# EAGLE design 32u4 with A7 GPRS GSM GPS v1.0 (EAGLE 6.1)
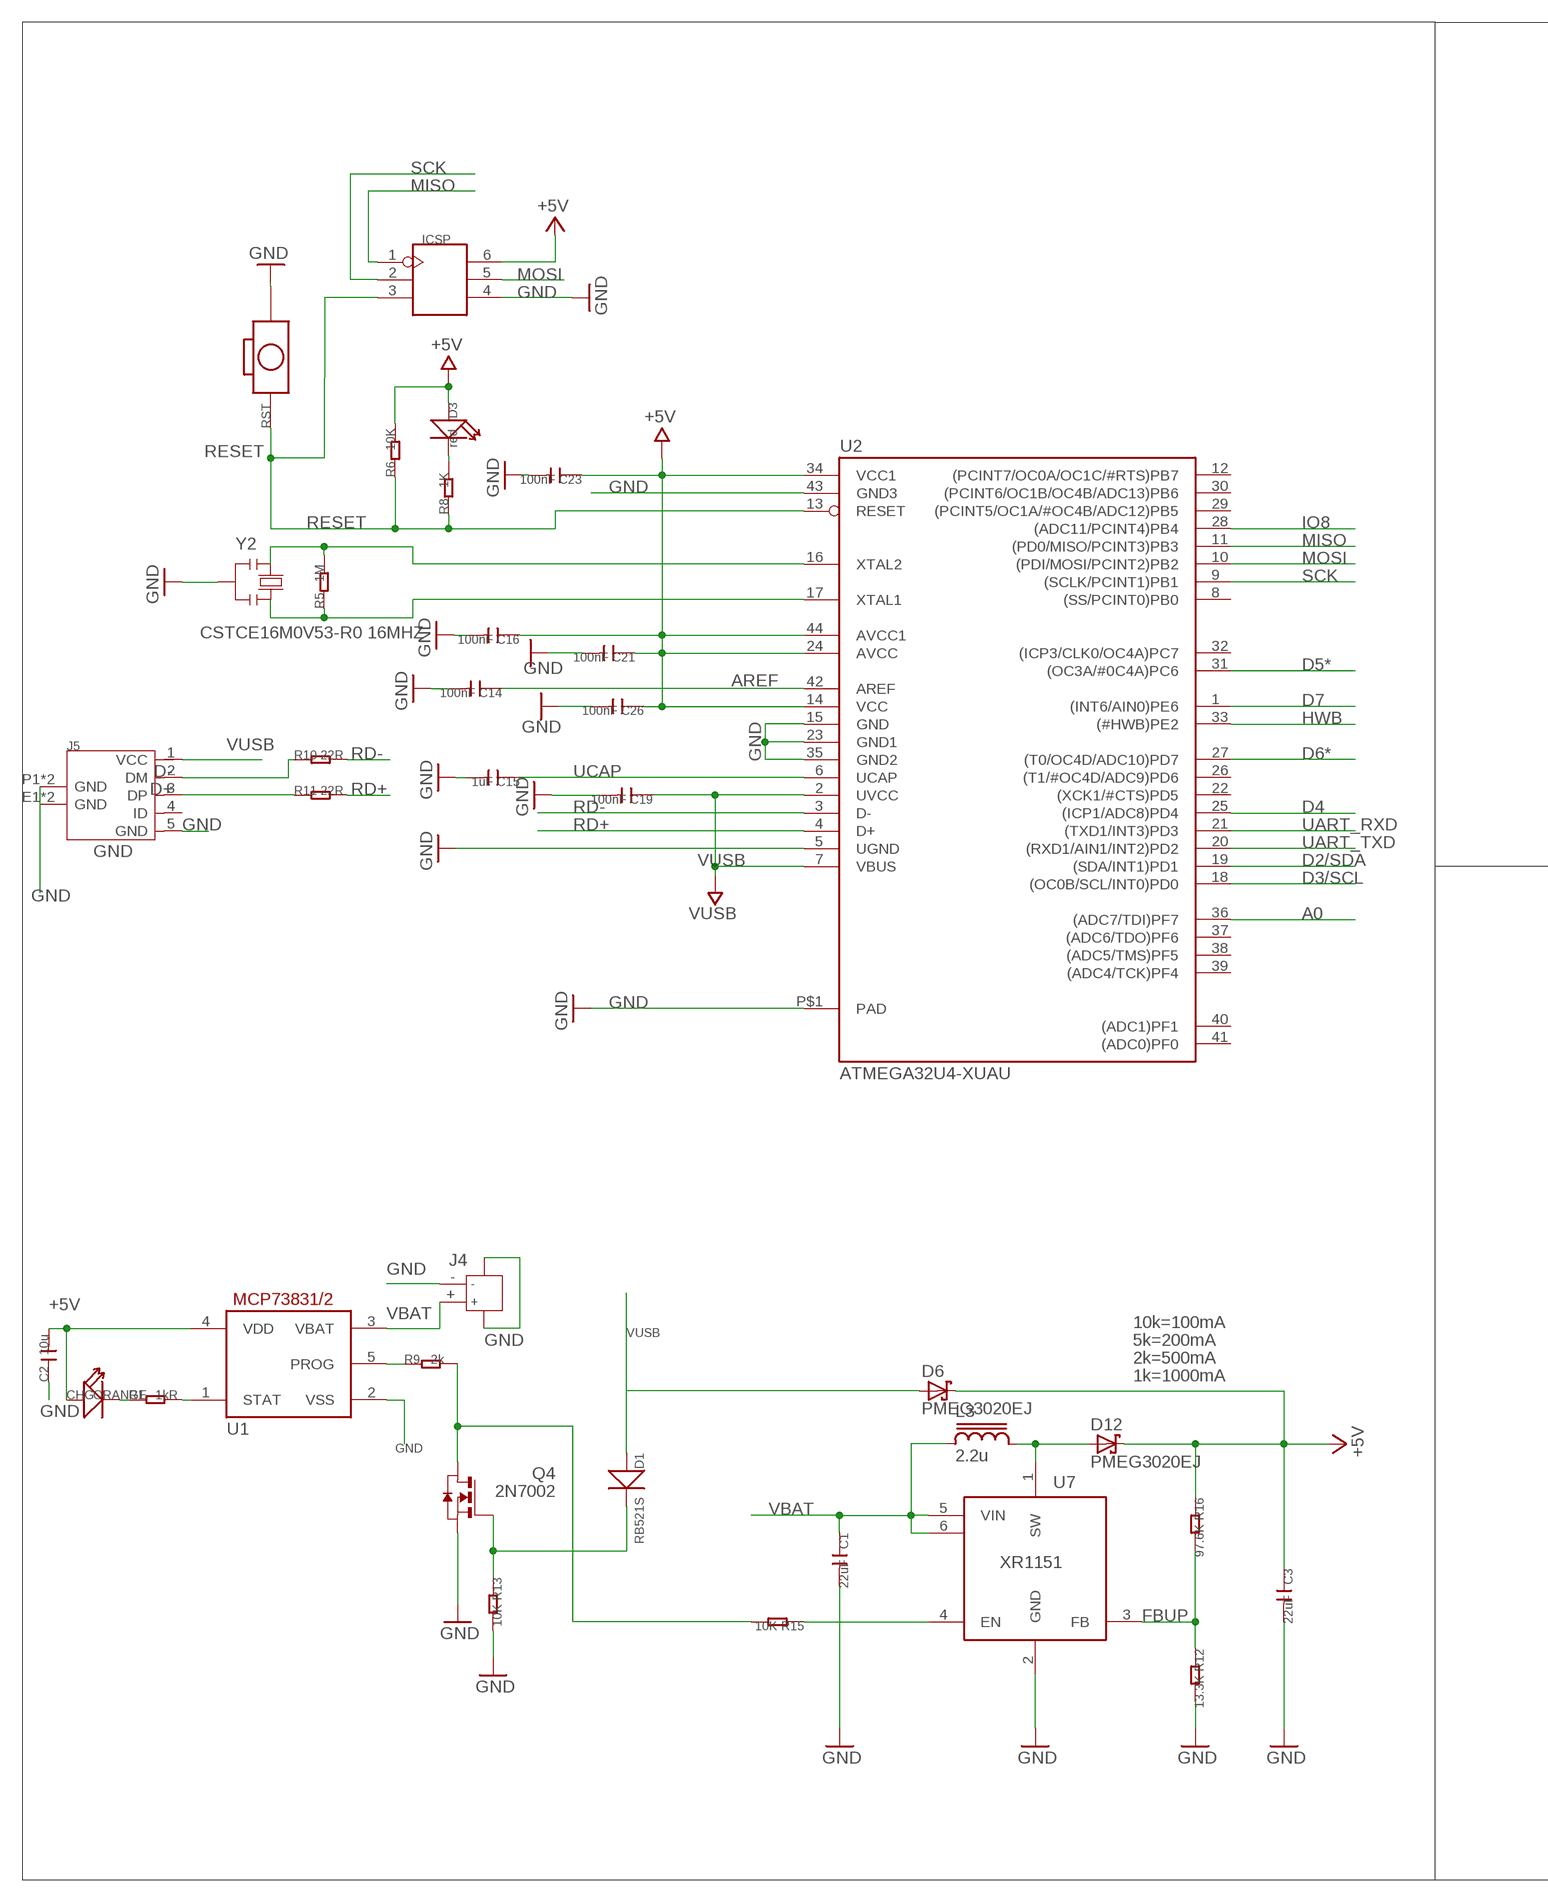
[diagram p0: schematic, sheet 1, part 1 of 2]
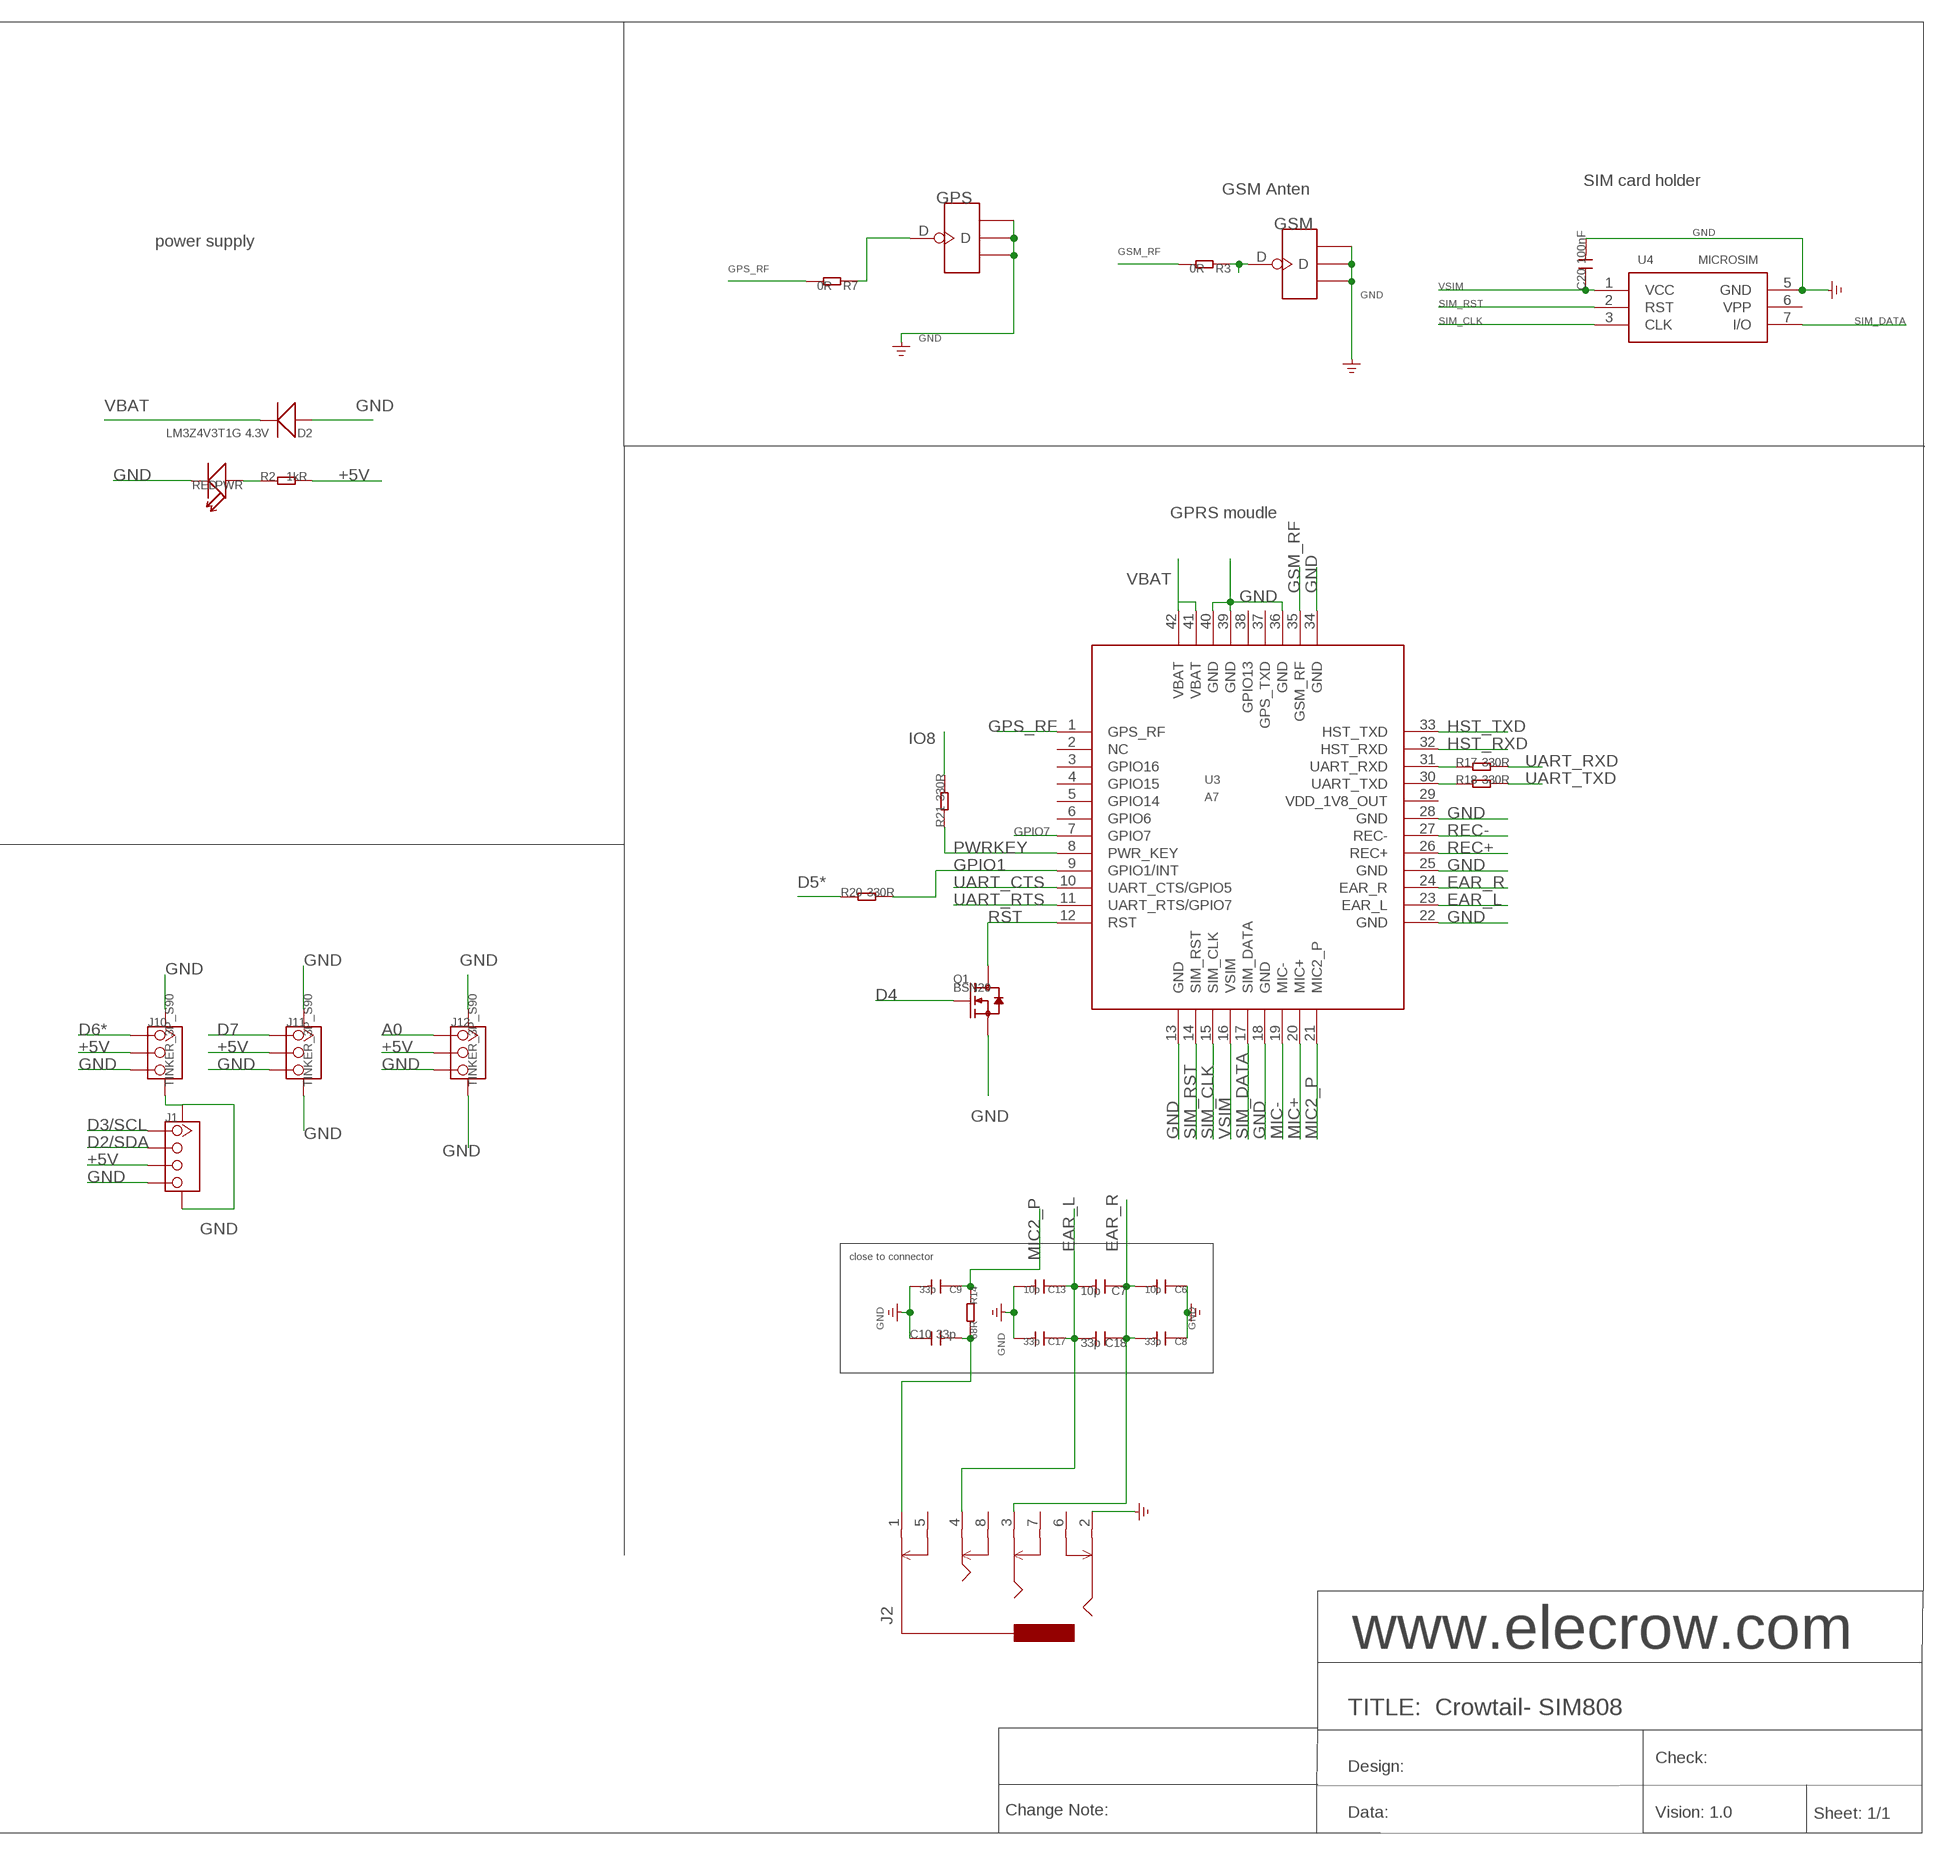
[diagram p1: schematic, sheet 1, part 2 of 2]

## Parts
C1  22uF  C-0603  [C0603]
C2  10u  C-0603  [C0603]
C3  22uF  C-0603  [C0603]
C6  10p  C-0402  [C0402]
C7  10p  C-0402  [C0402]
C8  33p  C-0402  [C0402]
C9  33p  C-0603  [C0603]
C10  33p  C-0603  [C0603]
C13  10p  C-0402  [C0402]
C14  100nF  C-0603  [C0603]
C15  1uF  C-0603  [C0603]
C16  100nF  C-0603  [C0603]
C17  33p  C-0402  [C0402]
C18  33p  C-0402  [C0402]
C19  100nF  C-0603  [C0603]
C20  100nF  C-0603  [C0603]
C21  100nF  C-0603  [C0603]
C23  100nF  C-0603  [C0603]
C26  100nF  C-0603  [C0603]
CHG  ORANGE  007-LED0603  [D0603]
D1  RB521S  D'0603'  [SOD523]
D2  LM3Z4V3T1G 4.3V  D'0805'  [SOD323]
D3  red  LED'0603'  [LED-0603]
D6  PMEG3020EJ  [SOD-323]
D12  PMEG3020EJ  [SOD-323]
GPS  ANTENNA-U-FL  [4P-U-FL]
GSM  ANTENNA-U-FL  [4P-U-FL]
ICSP  HEADER-2X3P-2.0  [2X3P-2.0]
J1  TWIG-4P-2.0-SMD-FEMALE-REINFORCE'90D'  [4P-SMD-2.0-90D]
J2  AUDIO-8P'PJ-3536-L6S'  [8P-3.5-SMD]
J4  JACK-JST-2P-SMD-PW'2.0'  [JST-SMD-2.0-90D]
J5  MICRO-USB-5P-340015001  [B-SMD-5P]
J10  TINKER_3P_S90  [TINKER_3P_S90]
J11  TINKER_3P_S90  [TINKER_3P_S90]
J12  TINKER_3P_S90  [TINKER_3P_S90]
L3  2.2u  LCD32  [CD32]
PWR  RED  007-LED0603  [D0603]
Q1  BSN20  MOSFET-N'SOT23'  [SOT23@1]
Q4  2N7002  [SOT23]
R1  1kR  R-0603  [R0603]
R2  1kR  R-0603  [R0603]
R3  0R  R-0603  [R0603]
R5  1M  R-0603  [R0603]
R6  10K  R-0603  [R0603]
R7  0R  R-0603  [R0603]
R8  1K  R-0603  [R0603]
R9  2k  R-0603  [R0603]
R10  22R  R-0603  [R0603]
R11  22R  R-0603  [R0603]
R12  13.3K  R-0603  [R0603]
R13  10K  R-0603  [R0603]
R14  68R  R-0603  [R0603]
R15  10K  R-0603  [R0603]
R16  97.6K  R-0603  [R0603]
R17  330R  R-0603  [R0603]
R18  330R  R-0603  [R0603]
R20  330R  R-0603  [R0603]
R21  330R  R-0603  [R0603]
RST  BOTTON-2P-90D  [2P-7.62X3.56-90D]
U1  MCP73831/OT  [SOT23-5L]
U2  ATMEGA32U4-XUAU  [TQFP44-PAD]
U3  A7  [A7]
U4  MICROSIM  [MICROSIM]
U7  XR1151  [SOT23-6L]
Y2  CSTCE16M0V53-R0 16MHZ  RESONATORMU  [RESONATOR]

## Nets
+5V: C2.2 C3.1 C16.1 C21.1 C23.1 C26.1 CHG.+ D3.+ D6.C D12.C ICSP.6 J1.3 J10.2 J11.2 J12.2 R2.2 R6.2 R16.1 U1.4(VDD) U2.14(VCC) U2.24(AVCC) U2.34(VCC1) U2.44(AVCC1)
A0: J12.1 U2.36((ADC7/TDI)PF7)
AREF [aref]: C14.1 U2.42(AREF)
D2/SDA: J1.2 U2.19((SDA/INT1)PD1)
D3/SCL: J1.1 U2.18((OC0B/SCL/INT0)PD0)
D4: Q1.1(G) U2.25((ICP1/ADC8)PD4)
D5*: R20.1 U2.31((OC3A/#0C4A)PC6)
D6*: J10.1 U2.27((T0/OC4D/ADC10)PD7)
D7: J11.1 U2.1((INT6/AIN0)PE6)
D+: J5.3(DP) R11.1
D-: J5.2(DM) R10.1
EAR_L: C7.2 C13.1 C17.1 C18.2 J2.4 U3.23(EAR_L)
EAR_R: C6.2 C7.1 C8.2 C18.1 J2.3 U3.24(EAR_R)
FBUP: R12.1 R16.2 U7.3(FB)
GND: C1.2 C2.1 C3.2 C6.1 C8.1 C9.2 C10.1 C13.2 C14.2 C15.2 C16.2 C17.2 C19.2 C20.2 C21.2 C23.2 C26.2 D2.+ GPS.GND1 GPS.GND2 GPS.GND3 GSM.GND1 GSM.GND2 GSM.GND3 ICSP.4 J1.4 J1.SS1 J1.SS2 J2.2 J4.3 J4.4 J4.- J5.5(GND) J5.E1(GND) J5.E2(GND) J5.P1(GND) J5.P2(GND) J10.3 J10.SS1 J10.SS2 J11.3 J11.SS1 J11.SS2 J12.3 J12.SS1 J12.SS2 PWR.- Q1.2(S) Q4.2(S) R12.2 R13.2 RST.P$2 U1.2(VSS) U2.5(UGND) U2.15(GND) U2.23(GND1) U2.35(GND2) U2.43(GND3) U2.P$1(PAD) U3.13(GND) U3.18(GND) U3.22(GND) U3.25(GND) U3.28(GND) U3.34(GND) U3.36(GND) U3.39(GND) U3.40(GND) U4.5(GND) U7.2(GND) Y2.2
GPIO1: R20.2 U3.9(GPIO1/INT)
GPIO7: U3.7(GPIO7)
GPS_RF: R7.2 U3.1(GPS_RF)
GSM_RF: R3.2 U3.35(GSM_RF)
HST_RXD: U3.32(HST_RXD)
HST_TXD: U3.33(HST_TXD)
HWB: U2.33((#HWB)PE2)
IO8: R21.2 U2.28((ADC11/PCINT4)PB4)
MIC2_P: C9.1 R14.1 U3.21(MIC2_P)
MIC+: U3.20(MIC+)
MIC-: U3.19(MIC-)
MISO: ICSP.1 U2.11((PD0/MISO/PCINT3)PB3)
MOSI: ICSP.5 U2.10((PDI/MOSI/PCINT2)PB2)
N$1: D12.A L3.2 U7.1(SW)
N$2: Q4.3(D) R9.2 R15.2
N$3: D1.- Q4.1(G) R13.1
N$4: R17.1 U3.31(UART_RXD)
N$5: GSM.D R3.1
N$6: PWR.+ R2.1
N$7: GPS.D R7.1
N$10: R15.1 U7.4(EN)
N$11: CHG.- R1.1
N$14: R18.1 U3.30(UART_TXD)
N$15: D3.- R8.2
N$20: R1.2 U1.1(STAT)
N$30: C10.2 J2.1 R14.2
N$31: R9.1 U1.5(PROG)
PWRKEY: R21.1 U3.8(PWR_KEY)
RD+: R11.2 U2.4(D+)
RD-: R10.2 U2.3(D-)
REC+: U3.26(REC+)
REC-: U3.27(REC-)
RESET: ICSP.3 R6.1 R8.1 RST.P$1 U2.13(RESET)
RST: Q1.3(D) U3.12(RST)
SCK: ICSP.2 U2.9((SCLK/PCINT1)PB1)
SIM_CLK: U3.15(SIM_CLK) U4.3(CLK)
SIM_DATA: U3.17(SIM_DATA) U4.7(I/O)
SIM_RST: U3.14(SIM_RST) U4.2(RST)
UART_CTS: U3.10(UART_CTS/GPIO5)
UART_RTS: U3.11(UART_RTS/GPIO7)
UART_RXD: R17.2 U2.21((TXD1/INT3)PD3)
UART_TXD: R18.2 U2.20((RXD1/AIN1/INT2)PD2)
UCAP: C15.1 U2.6(UCAP)
VBAT: C1.1 D2.- J4.+ L3.1 U1.3(VBAT) U3.41(VBAT) U3.42(VBAT) U7.5(VIN) U7.6(VIN1)
VSIM: C20.1 U3.16(VSIM) U4.1(VCC)
VUSB: C19.1 D1.+ D6.A J5.1(VCC) U2.2(UVCC) U2.7(VBUS)
XTAL3: R5.2 U2.16(XTAL2) Y2.1
XTAL4: R5.1 U2.17(XTAL1) Y2.3
Unconnected: J2.5 J2.6 J2.7 J2.8 J5.4(ID) U2.8((SS/PCINT0)PB0) U2.12((PCINT7/OC0A/OC1C/#RTS)PB7) U2.22((XCK1/#CTS)PD5) U2.26((T1/#OC4D/ADC9)PD6) U2.29((PCINT5/OC1A/#OC4B/ADC12)PB5) U2.30((PCINT6/OC1B/OC4B/ADC13)PB6) U2.32((ICP3/CLK0/OC4A)PC7) U2.37((ADC6/TDO)PF6) U2.38((ADC5/TMS)PF5) U2.39((ADC4/TCK)PF4) U2.40((ADC1)PF1) U2.41((ADC0)PF0) U3.2(NC) U3.3(GPIO16) U3.4(GPIO15) U3.5(GPIO14) U3.6(GPIO6) U3.29(VDD_1V8_OUT) U3.37(GPS_TXD) U3.38(GPIO13) U4.6(VPP)

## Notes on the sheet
- SIM card holder
- GSM Anten
- power supply
- GPRS moudle
- close to connector
- 10k=100mA
- 5k=200mA
- 2k=500mA
- 1k=1000mA
- www.elecrow.com
- TITLE:  Crowtail- SIM808
- Check:
- Design:
- Change Note: | Data: | Vision: 1.0 | Sheet: 1/1

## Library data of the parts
C1-C3 C6-C10 C13-C21 C23 C26 = Discrete:C*: Ceramic Capacitors
CHG PWR = Discrete:007-LED*
D1 D2 = Discrete:D*
D3 = Discrete:LED*
D6 D12 = Max-Diodes:PMEG3020
GPS GSM = Connector:ANTENNA-U-FL
ICSP = Connector:HEADER-2X3P
J1 = Connector:TWIG-4P-2.0-SMD-FEMALE-REINFORCE
J2 = template:AUDIO-8P
J4 = Connector:JACK-JST-2P-SMD-PW
J5 = OPL Eagle Library:MICRO-USB-5P: ST-USB-001E：MICRO USB B SMD R/A
J10-J12 = Connector:TINKER_3P_S90
L3 = Max-RCL:L
Q1 = Discrete:MOSFET-N: IRLL014: http://www.vishay.com/docs/91319/sihll014.pdf
Q4 = Max-Mosfets:2N7002
R1-R3 R5-R18 R20 R21 = Discrete:R*
RST = Discrete:BOTTON-2P
U1 = adafruit:MCP73831: MCP73831/2 Miniature Single-Cell, Fully Integrated Li-Ion, Li-Polymer Charge Management Controllers. Nice and small simple lipoly charge controller, with adjustable current and status output (LED) http://www.ladyada.net/library/pcb/eaglelibrary.html
U2 = SmartPrj:ATMEGA32U4-XU
U3 = IC:A7
U4 = Connector:MICROSIM
U7 = Max-SwitchingRegulators:XR1151
Y2 = SmartPrj:RESONATOR

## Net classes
0 default: width 0.152 mm, drill 0.152 mm, clearance 0.152 mm
1 power: width 0.61 mm, drill 0.61 mm, clearance 0.203 mm
2 gnd: width 0.305 mm, drill 0.559 mm, clearance 0.203 mm
3 usbvcc: width 0.508 mm, drill 0.61 mm, clearance 0.203 mm
4 aref: width 0.254 mm, drill 0.61 mm, clearance 0.254 mm

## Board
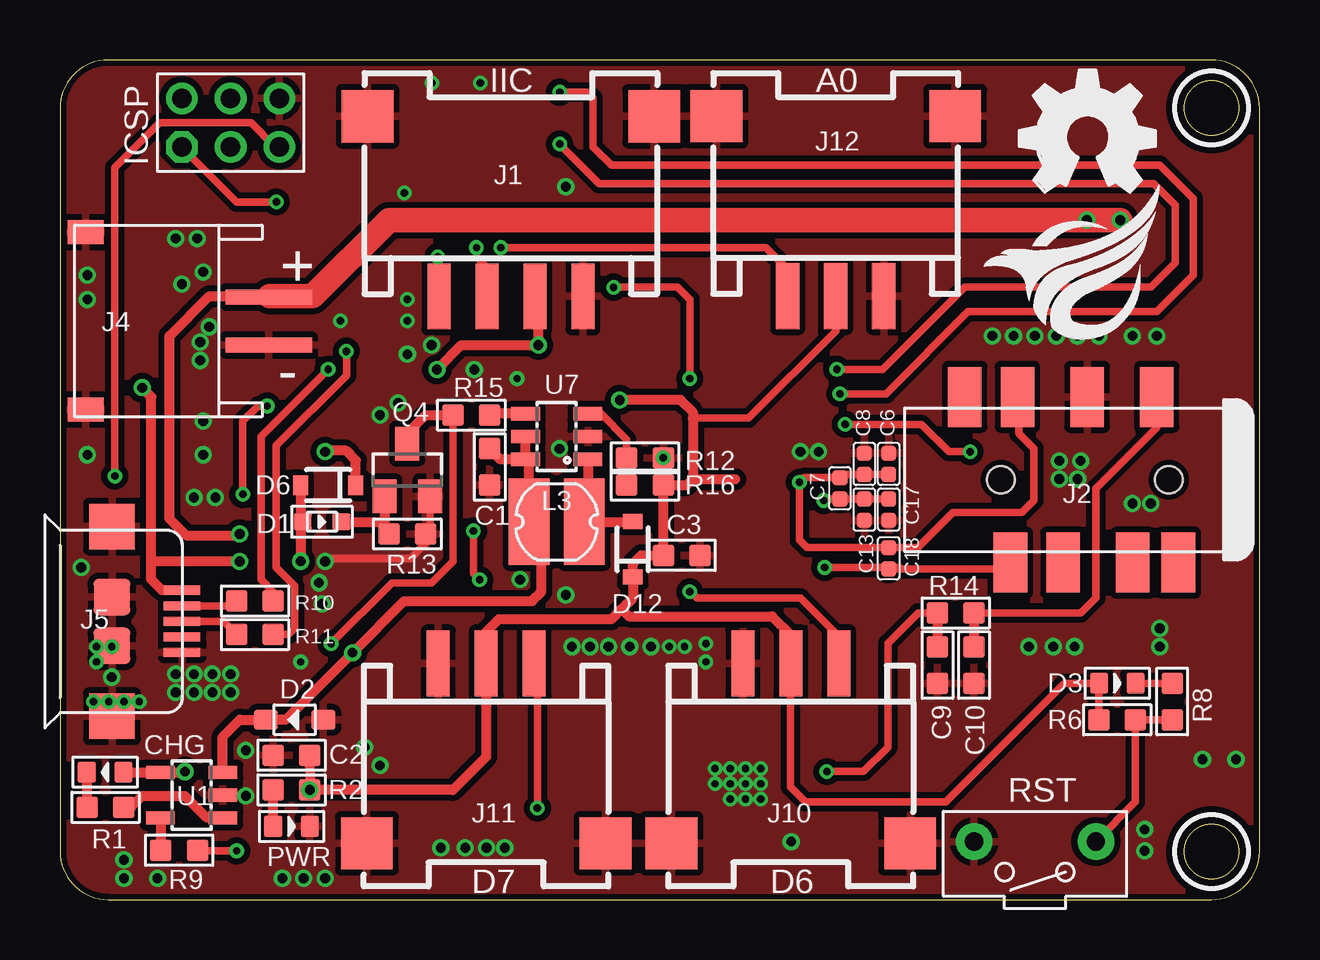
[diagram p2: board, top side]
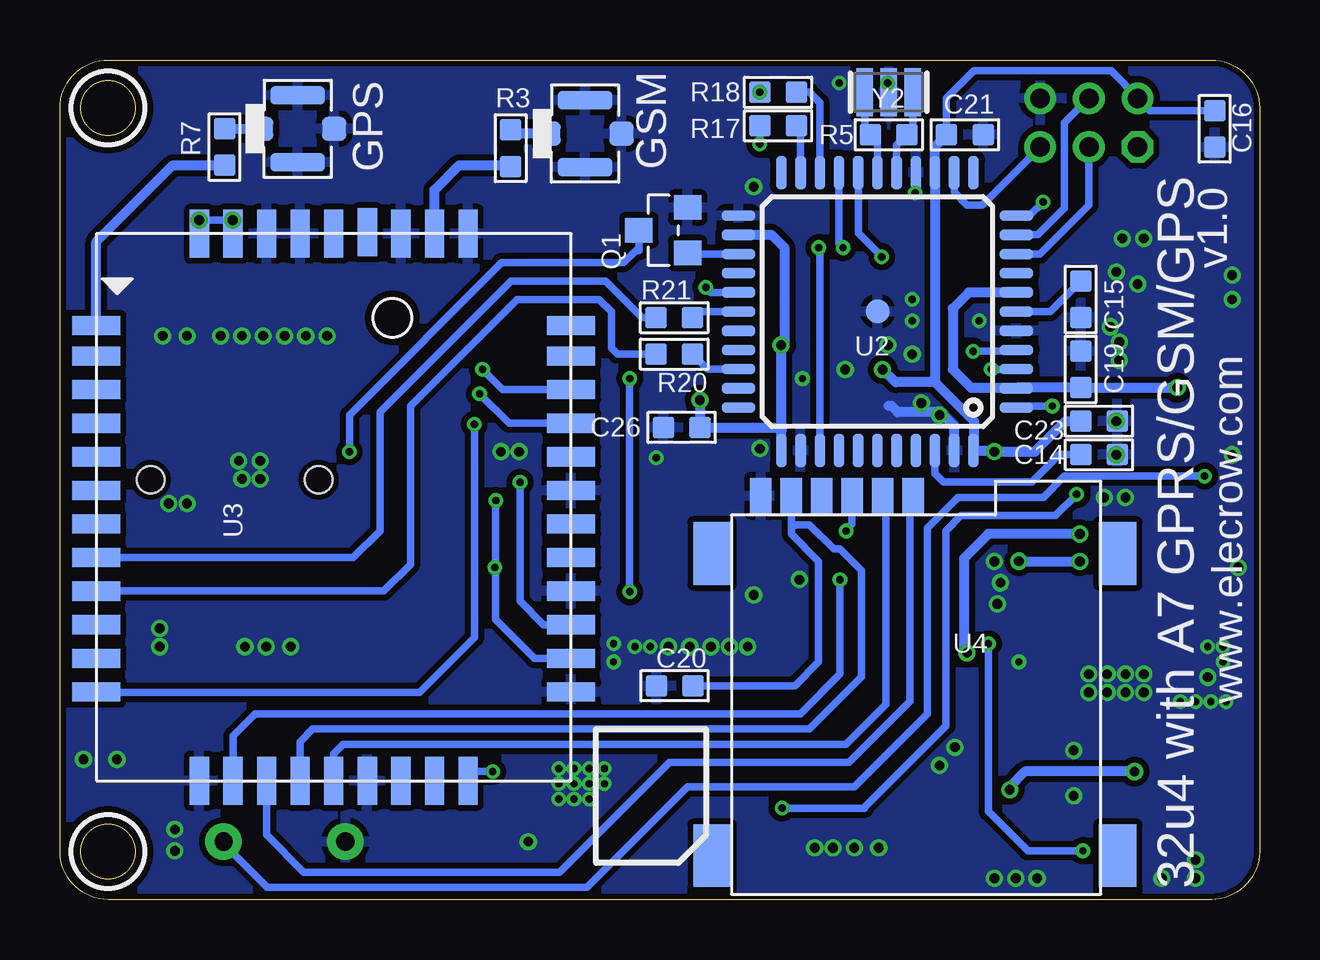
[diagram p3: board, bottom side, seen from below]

Size 50 x 35 mm. Coordinates in mm from the lower left corner, seen from the top.
Outline: 0,33 0,2 arc90 2,0 48,0 arc90 50,2 50,33 arc90 48,35 2,35 arc90 0,33
Outline: circle at 48,2 radius 1.14
Outline: circle at 48,33 radius 1.14
Copper layers (1*16): Top 0.035mm / dielectric 1.5mm / Bottom 0.035mm
Design rules: minimum track width 6mil, minimum drill 12mil, track to track 6mil, track to pad 6mil, pad to pad 6mil, via to via 6mil, smd to smd 0mil, copper to edge 10mil, drill to drill 10mil, minimum pad ring 10mil, minimum via ring 6mil, stop-mask expansion 2mil, vias tented up to drill 100mil, thermal gap 10mil
tRestrict: area 35.6,41.9 to 35.7,43.3; area 46.5,0.5 to 49.5,3.5; area 46.5,31.5 to 49.5,34.5
bRestrict: area 46.5,0.5 to 49.5,3.5; area 46.5,31.5 to 49.5,34.5

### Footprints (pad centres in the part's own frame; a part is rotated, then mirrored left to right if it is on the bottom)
C0603 = smd 0.889 x 0.889: 1 -0.762,0; 2 0.762,0
C0402 = smd 0.635 x 0.635: 1 -0.445,0; 2 0.445,0
D0603 = smd 0.762 x 0.889: + -0.762,0; - 0.762,0
SOD523 = smd 0.762 x 0.7: + -0.8,0; - 0.8,0
SOD323 = smd 1 x 0.8: + -1.2,0; - 1.2,0
LED-0603 = smd 0.762 x 0.889: + -0.762,0; - 0.762,0
SOD-323 = smd 0.63 x 0.83: A 1.15,0; C -1.15,0
4P-U-FL = smd 1.016 x 1.016: D -1.524,0; GND3 1.524,0 | smd 2.286 x 0.762: GND1 0,1.397; GND2 0,-1.397
2X3P-2.0 = drill 0.813 pad 1.27 octagon: 1 -1.016,2.032 | drill 0.813 pad 1.27: 2 -1.016,0; 3 -1.016,-2.032; 4 1.016,-2.032; 5 1.016,0; 6 1.016,2.032
4P-SMD-2.0-90D = smd 0.965 x 2.74: 1 -3,-0.1; 2 -1,-0.1; 3 1,-0.1; 4 3,-0.1 | smd 2.159 x 2.184: SS1 -5.974,7.4; SS2 5.974,7.4
8P-3.5-SMD = smd 1.4 x 2.5: 1 2.8,-3.45; 2 5.7,-3.45; 3 8.6,-3.45; 4 8.9,3.45; 5 1.9,3.45; 6 3.8,3.45; 7 6.7,3.45; 8 10.8,-3.45 | hole 1.149: 2.3,0; 9.3,0
JST-SMD-2.0-90D = smd 1 x 1.5: 3 3.7,-2.54; 4 -3.7,-2.54 | smd 0.635 x 3.6: + -1,5.08; - 1,5.08
B-SMD-5P = smd 0.38 x 1.52: 1 -1.3,2.54; 2 -0.65,2.54; 3 0,2.54; 4 0.65,2.54; 5 1.3,2.54 | smd 1.524 x 1.524: E1 -1.016,-0.381; E2 1.016,-0.381 | smd 1.9 x 1.9: P1 -3.95,-0.381; P2 3.95,-0.381
TINKER_3P_S90 = smd 0.965 x 2.74: 1 -1.984,-4.545; 2 0.016,-4.545; 3 2.016,-4.545 | smd 2.159 x 2.184: SS1 -4.958,2.955; SS2 4.99,2.955
CD32 = smd 3.6 x 1.7: 1 0,1.15; 2 0,-1.15
SOT23@1 = smd 1.016 x 1.143: 1 -0.95,-1.016; 2 0.95,-1.016; 3 0,1.016
SOT23 = smd 1 x 1.4: 1 -0.95,-1.1; 2 0.95,-1.1; 3 0,1.1
R0603 = smd 0.889 x 0.889: 1 -0.762,0; 2 0.762,0
2P-7.62X3.56-90D = drill 0.762 pad 1.524: P$1 0,2.54; P$2 0,-2.54
SOT23-5L = smd 0.55 x 1.2: 1 -0.95,-1.3; 2 0,-1.3; 3 0.95,-1.3; 4 0.95,1.3; 5 -0.95,1.3
TQFP44-PAD = smd 1.4 x 0.45: 1 -5.8,4; 2 -5.8,3.2; 3 -5.8,2.4; 4 -5.8,1.6; 5 -5.8,0.8; 6 -5.8,0; 7 -5.8,-0.8; 8 -5.8,-1.6; 9 -5.8,-2.4; 10 -5.8,-3.2; 11 -5.8,-4; 23 5.8,-4; 24 5.8,-3.2; 25 5.8,-2.4; 26 5.8,-1.6; 27 5.8,-0.8; 28 5.8,0; 29 5.8,0.8; 30 5.8,1.6; 31 5.8,2.4; 32 5.8,3.2; 33 5.8,4 | smd 0.45 x 1.4: 12 -4,-5.8; 13 -3.2,-5.8; 14 -2.4,-5.8; 15 -1.6,-5.8; 16 -0.8,-5.8; 17 0,-5.8; 18 0.8,-5.8; 19 1.6,-5.8; 20 2.4,-5.8; 21 3.2,-5.8; 22 4,-5.8; 34 4,5.8; 35 3.2,5.8; 36 2.4,5.8; 37 1.6,5.8; 38 0.8,5.8; 39 0,5.8; 40 -0.8,5.8; 41 -1.6,5.8; 42 -2.4,5.8; 43 -3.2,5.8; 44 -4,5.8 | smd 1 x 1: P$1 0,0
A7 = smd 0.8 x 2: 1 7.57,9.9; 2 6.3,9.9; 3 4.9,9.9; 4 3.5,9.9; 5 2.1,9.9; 6 0.7,9.9; 7 -0.7,9.9; 8 -2.1,9.9; 9 -3.5,9.9; 10 -4.9,9.9; 11 -6.3,9.9; 12 -7.7,9.9; 22 -7.7,-9.9; 23 -6.3,-9.9; 24 -4.9,-9.9; 25 -3.5,-9.9; 26 -2.1,-9.9; 27 -0.7,-9.9; 28 0.7,-9.9; 29 2.1,-9.9; 30 3.5,-9.9; 31 4.9,-9.9; 32 6.3,-9.9; 33 7.57,-9.9 | smd 2 x 0.8: 13 -11.4,5.6; 14 -11.4,4.2; 15 -11.4,2.8; 16 -11.4,1.4; 17 -11.4,0; 18 -11.4,-1.4; 19 -11.4,-2.8; 20 -11.4,-4.2; 21 -11.4,-5.6; 34 11.4,-5.6; 35 11.4,-4.2; 36 11.4,-2.8; 37 11.46,-1.4; 38 11.4,0; 39 11.4,1.4; 40 11.4,2.8; 41 11.4,4.2; 42 11.4,5.6
MICROSIM = smd 1.5 x 0.9: 1 -0.8,2.5; 2 -0.8,5.04; 3 -0.8,7.58; 5 -0.8,1.23; 6 -0.8,3.77; 7 -0.8,6.31 | smd 2.61 x 1.56: P$1 1.6,-0.8; P$2 14.2,-0.8; P$3 14.2,16.1; P$4 1.6,16.1
SOT23-6L = smd 0.55 x 1.2: 1 -0.95,-1.3; 2 0,-1.3; 3 0.95,-1.3; 4 0.95,1.3; 5 0,1.3; 6 -0.95,1.3
RESONATOR = smd 0.7 x 2: 1 -1,0; 2 0,0; 3 1,0

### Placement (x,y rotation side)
C1  17.91,18.03 270 top
C2  9.65,6.02 0 top
C3  25.91,14.35 0 top
C6  34.54,18.16 270 top
C7  32.51,17.14 270 top
C8  33.53,18.16 270 top
C9  36.58,9.78 270 top
C10  38.1,9.78 90 top
C13  33.53,16.26 270 top
C14  6.69,18.54 0 bottom
C15  7.46,25.02 270 bottom
C16  1.87,32.13 270 bottom
C17  34.54,16.26 270 top
C18  34.54,14.22 270 top
C19  7.46,22.1 90 bottom
C20  24.38,8.91 180 bottom
C21  12.28,31.88 0 bottom
C23  6.69,19.94 0 bottom
C26  24.09,19.68 180 bottom
CHG  1.88,5.31 180 top
D1  10.92,15.75 0 top
D2  9.78,7.49 180 top
D3  44.07,9.02 0 top
D6  11.18,17.27 180 top
D12  23.88,14.61 90 top
GPS  40.09,32.13 0 bottom
GSM  28.11,31.93 0 bottom
ICSP  7.11,32.38 90 top
J1  18.8,25.25 0 top
J2  48.51,17.5 180 top
J4  3.62,24.12 270 top
J5  2.55,11.6 270 top
J10  30.48,5.3 180 top
J11  17.78,5.3 180 top
J12  32.32,29.7 0 top
L3  20.7,15.75 90 top
LOGO2  LOGO-OSHW-FILLX0200-NT  [OSHW_FILLX200_NOTEXT]  39.99,29.5 0 top
PWR  9.65,3.05 0 top
Q1  24.85,27.9 90 bottom
Q4  14.48,17.91 0 top
R1  1.9,3.84 0 top
R2  9.65,4.57 0 top
R3  31.21,31.32 270 bottom
R5  15.46,31.88 0 bottom
R6  44.07,7.49 180 top
R7  43.14,31.37 270 bottom
R8  46.35,8.26 90 top
R9  4.97,2.06 0 top
R10  8.13,12.45 0 top
R11  8.13,11.05 0 top
R12  24.38,18.41 0 top
R13  14.48,15.24 0 top
R14  37.34,11.94 0 top
R15  17.14,20.19 180 top
R16  24.38,17.27 180 top
R17  20.07,32.26 0 bottom
R18  20.07,33.66 0 bottom
R20  24.4,22.73 180 bottom
R21  24.4,24.26 0 bottom
RST  40.64,2.41 270 top
U1  5.49,4.36 90 top
U2  15.93,24.51 180 bottom
U3  38.59,16.36 90 bottom
U4  22.01,16.03 270 bottom
U7  20.7,19.3 90 top
U$4  [ELECROW_NRW_6]  38.5,23.35 0 top
Y2  15.46,33.66 180 bottom

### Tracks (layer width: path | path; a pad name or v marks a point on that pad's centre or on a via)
+5V  (via drill 0.41)
  Top 0.305: R6.2 D3.+ 41.87,9.02 36.92,4.06 31.08,4.06 30.44,4.7 30.44,9.82 J10.2 | J12.2 32.34,23.7 28.7,20.07 26.38,20.07
  Top 0.406: 23.41,12.11 23.88,12.57 D12.C 23.88,14.01 24.22,14.35 C3.1 R16.1 26.12,17.27 26.38,17.53 | 23.41,12.11 22.99,11.68 18.29,11.68 17.76,11.16 J11.2 17.76,5.95 16.38,4.57 R2.2 10.44,4.59 C2.2 | 32.35,25.14 J12.2 | J10.2 30.53,9.78 30.57,9.78 30.44,9.91 30.44,11.05 29.68,11.81 23.71,11.81 23.41,12.11 | v15.71,22.1 16.73,23.11 v19.94,23.11 19.94,25.01 J1.3 | 11.11,18.61 v11.05,18.67 11.09,18.71 U2.44 12.33,18.31 D6.C | CHG.+ U1.4 5.18,5.31 v5.21,5.33 | 26.38,17.53 26.38,20.07 26.38,20.32 25.87,20.83 v23.33,20.83 | 26.38,17.53 28.16,17.53
  Bottom 0.305: C16.1 4.57,32.89 ICSP.6 5.04,33.4 6.18,34.54 11.9,34.54 13.04,33.4 C21.1
  Bottom 0.406: U2.34 19.93,19.56 | C21.1 13.53,31.39 U2.14 13.53,21.57 | 13.53,21.57 11.9,19.94 11.9,18.74 U2.44 11.09,18.71 v11.05,18.67 9.36,18.67 8.09,19.94 C23.1 | 13.53,21.57 15.18,21.57 v15.71,22.1 | 19.93,19.56 20.05,19.68 C26.1 v23.33,20.83 | 19.93,19.56 19.93,23.1 v19.94,23.11 19.81,23.24 19.81,27.18 20.34,27.71 U2.24 | v5.21,5.33 9.78,5.33 10.41,4.7 R2.2
  other vias: 10.41,4.57
A0  (via drill 0.3)
  Top 0.305: v18.38,27.18 29.43,27.18 30.44,26.16 30.44,25.15 30.32,25.27
  Top 0.406: 30.48,25.27 30.36,25.16 J12.1 30.34,25.15 30.44,25.15
  Bottom 0.305: U2.36 18.33,27.13 v18.38,27.18
AREF
  Bottom 0.305: C14.1 8.34,18.54 9.49,17.4 13.17,17.4 13.53,17.75 U2.42
D2/SDA  (via drill 0.3)
  Top 0.305: v17.36,27.18 17.36,26.8 17.74,26.42 17.74,25.4 18,25.15 J1.2 | 17.74,25.15 J1.2 | J1.2
  Bottom 0.305: U2.19 17.53,27.34 v17.36,27.18
D3/SCL  (via drill 0.3)
  Top 0.406: v15.75,26.8 15.75,25.2 J1.1
  Bottom 0.305: U2.18 16.73,27.77 v15.75,26.8
D4
  Bottom 0.305: U2.25 23.8,26.91 Q1.1
D5*
  Bottom 0.305: U2.31 23.01,22.11 R20.1
D6*  (via drill 0.3)
  Top 0.305: v23.08,25.53 25.74,25.53 26.25,25.02 v26.25,21.72 | J10.1 32.47,9.86 32.47,10.88 32.51,10.92 30.86,12.57 26.54,12.57 26.29,12.83 v26.25,12.83
  Bottom 0.305: U2.27 22.86,25.31 v23.08,25.53 | v26.25,21.72 v26.25,12.83
D7  (via drill 0.3)
  Top 0.305: v19.9,3.81 19.9,9.71 J11.1 | v7.62,16.89 7.62,19.94 8.26,20.57 v8.64,20.57
  Bottom 0.305: v19.9,3.81 16.47,3.81 16.47,3.85 13.08,7.24 13.08,15.37 12.45,16 8.51,16 v7.62,16.89 | v8.64,20.57 10.06,20.57 U2.1
D+
  Top 0.305: J5.3 6.82,11.6 R11.1
D-
  Top 0.305: J5.2 7.17,12.24 R10.1
EAR_L  (via drill 0.3)
  Top 0.305: C17.1 C13.1 C7.2 31.9,16.7 v31.84,16.64 | C18.2 35.05,13.78 | 35.05,13.78 39.34,13.78 J2.4 | v31.88,13.84 34.99,13.84 35.05,13.78
  Bottom 0.305: v31.84,16.64 31.84,13.84 | 31.84,13.84 31.84,11.68 30.21,10.06 U3.23 | v31.88,13.84 31.84,13.84
EAR_R  (via drill 0.3)
  Top 0.305: C6.2 C8.2 32.51,17.72 C7.1 31.01,17.59 v30.82,17.4 30.82,14.99 31.14,14.67 C18.1 35.75,14.67 37.21,16.13 40.09,16.13 40.6,16.64 40.6,18.8 39.97,19.43 39.97,20.9 J2.3
  Bottom 0.305: v30.82,17.4 30.82,12.45 29.83,11.46 U3.24
FBUP
  Top 0.305: U7.3 22.55,20.25 23.62,19.18 R12.1
  Top 0.406: R12.1 R16.2
GND  (via drill 0.3, 0.41)
  Top 0.305: v11.05,14.1 11.18,14.22 14.61,14.22 15.24,14.86 R13.2 15.43,15.43 Q4.2
  Bottom 0.406: Y2.2 15.46,34 v15.49,34.04 | U2.43 12.73,19.75 13.3,20.32 15.07,20.32 15.33,20.57 15.46,20.57 | U2.15 14.33,29.6 14.31,29.59 14.44,29.46 v14.35,29.46 14.31,29.46
  other vias: 14.48,25.02 14.48,24.13 11.68,24.13 19.05,21.72 26.92,10.67 26.92,9.91 10.03,9.91 2.16,10.54 21.08,29.72 17.53,34.04 40.39,10.54 41.4,10.54 17.78,2.16 16.89,2.16 10.16,0.89 9.27,0.89 4.83,8.64 6.35,9.4 5.08,25.65 1.14,18.54 5.71,27.56 4.83,27.56 14.48,22.73 45.72,23.5 43.31,23.5 41.66,18.29 17.27,22.1 14.1,20.7 45.85,11.3 24.64,10.54 23.75,10.54 0.89,13.84 1.14,25.02 5.59,8.64 7.11,9.4 12.7,6.35 30.48,2.41 2.67,0.89 4.06,0.89 13.34,5.59 6.48,16.76 5.84,23.24 5.84,22.48 5.97,18.54 5.97,19.94 5.97,26.16 10.79,13.21 6.35,8.64 7.75,4.32 18.54,2.16 45.85,10.54 42.29,10.54 47.62,5.84 49.02,5.84 42.55,18.29 44.7,16.51 44.7,23.5 45.21,2.92 45.21,2.03 6.22,23.88 7.11,8.64 25.15,18.41 19.18,13.34 22.86,10.54 21.08,12.7 13.34,20.19 20.83,18.8 15.49,23.11 7.75,6.22 15.88,2.16 5.59,16.76 1.14,26.04 5.59,9.4 4.83,9.4 10.92,12.32 2.16,9.27 2.67,1.65 11.05,0.89 41.66,17.53 42.42,17.53 45.47,16.51 42.42,23.5 41.53,23.5 40.64,23.5 39.75,23.5 38.86,23.5 30.86,18.67 31.62,18.67 25.4,10.54 26.04,10.54 22.1,10.54 21.34,10.54 27.3,5.46 27.94,5.46 28.57,5.46 29.21,5.46 29.21,4.83 29.21,4.19 28.57,4.19 28.57,4.83 27.94,4.83 27.94,4.19 27.3,4.83 1.52,10.54 1.52,9.91 1.4,8.26 2.03,8.26 2.67,8.26 3.3,8.26
  pour Bottom (isolate 0.254): -1.27,-1.27 50.8,-1.27 50.8,35.56 -1.27,35.56
  pour Top (isolate 0.254): -1.27,-1.27 50.8,-1.27 50.8,35.56 -1.27,35.56
GPIO1
  Bottom 0.305: R20.2 26.76,22.73 27.01,22.99 27.01,24.51 27.52,25.02 30.95,25.02 35.4,20.57 35.4,13.97 36.51,12.86 U3.9
GPS_RF
  Bottom 0.406: U3.1 48.49,27.42 45.3,30.61 R7.2
GSM_RF
  Bottom 0.406: U3.35 34.39,29.58 33.36,30.61 31.26,30.61 R3.2
IO8
  Bottom 0.305: U2.28 23.37,24.51 R21.2
MIC2_P  (via drill 0.3)
  Top 0.305: R14.1 35.78,11.94 34.51,10.67 34.51,6.35 33.49,5.33 v31.97,5.33
  Top 0.406: R14.1 C9.1
  Bottom 0.305: v31.97,5.33 32.61,5.33 U3.21
MISO  (via drill 0.3)
  Top 0.305: v9.02,29.08 7.37,29.08 ICSP.1
  Bottom 0.305: U2.11 9.59,28.51 v9.02,29.08
MOSI
  Bottom 0.305: U2.10 9.25,27.71 8.13,28.83 8.13,32.38 ICSP.5
N$1
  Top 0.406: D12.A 23.87,15.75 L3.2 22,15.9 U7.1
N$2  (via drill 0.3)
  Top 0.305: v7.37,2.03 5.75,2.03 R9.2 | R15.2 16.38,14.1 15.49,13.21 13.84,13.21 v11.3,10.67
  Top 0.406: Q4.3 14.48,19.43 15.24,20.19 16.26,20.19 16.38,20.32 R15.2
  Bottom 0.305: v7.37,2.03 9.65,2.03 11.3,3.68 v11.3,10.67
N$3
  Top 0.406: Q4.1 13.53,15.75 | 13.53,15.75 13.53,15.43 R13.1 | D1.- 13.53,15.75
N$4  (via drill 0.3)
  Top 0.305: v32.38,22.1 34.29,22.1 37.72,25.53 45.47,25.53 46.48,26.54 46.48,28.96 45.59,29.84 22.48,29.84 v20.83,31.5
  Bottom 0.305: U3.31 31.54,21.26 v32.38,22.1 | v20.83,31.5 R17.1 20.83,32.38
N$5
  Bottom 0.406: GSM.D 31.05,31.93 R3.1
N$6
  Top 0.406: PWR.+ R2.1
N$7
  Bottom 0.406: R7.1 GPS.D
N$10
  Top 0.406: U7.4 17.97,20.25 R15.1
N$11
  Top 0.406: CHG.- 1.12,3.86 R1.1
N$14  (via drill 0.3)
  Top 0.305: v32.51,21.08 34.42,21.08 37.85,24.51 45.72,24.51 47.24,26.04 47.24,29.21 45.85,30.61 22.99,30.61 22.23,31.37 22.23,33.4 21.97,33.66 R18.1
  Bottom 0.305: U3.30 31.29,19.86 v32.51,21.08
  other vias: 20.83,33.66
N$15
  Top 0.305: R8.2 D3.-
N$20
  Top 0.406: R1.2 2.95,3.84 3.43,4.32 5.21,4.32 6.1,3.43 6.77,3.43 U1.1
N$30
  Top 0.305: R14.2 42.55,11.94 43.18,12.57 43.18,17.14 45.72,19.68 J2.1
  Top 0.406: R14.2 C10.2
N$31
  Top 0.406: U1.5 4.19,2.29 4.32,2.16 R9.1
PWRKEY
  Bottom 0.305: R21.1 25.74,24.26 27.27,25.78 31.2,25.78 36.66,20.32 36.66,15.37 37.77,14.26 U3.8
RD+  (via drill 0.3)
  Top 0.305: R11.2 9.53,11.05 9.78,11.3 9.78,13.08 9.02,13.84 9.02,18.92 11.94,21.84 v11.94,22.86
  Bottom 0.305: v11.94,22.86 10.18,22.86 U2.4
RD-  (via drill 0.3)
  Top 0.305: R10.2 8.89,12.83 8.38,13.34 8.38,19.3 v11.18,22.1
  Bottom 0.305: v11.18,22.1 10.14,22.1 U2.3
RESET  (via drill 0.3)
  Top 0.305: R8.1 R6.1 44.83,4.06 RST.P$1 | ICSP.3 8.98,31.37 7.96,32.38 4.15,32.38 2.29,30.52 v2.29,17.65
  Bottom 0.305: U2.13 12.73,29.49 12.19,28.96 11.56,28.96 ICSP.3 | RST.P$1 43.27,2.41 41.36,0.51 28.03,0.51 23.84,4.7 16.89,4.7 13.84,7.75 13.84,15.49 12.57,16.76 9.02,16.76 8.13,17.65 v2.29,17.65
RST  (via drill 0.3)
  Top 0.305: v37.94,18.67 37.05,18.67 35.9,19.81 v32.73,19.81
  Bottom 0.305: Q1.3 25.87,27.05 26,27.05 26.5,26.54 31.59,26.54 37.94,20.19 v37.94,18.67 | v32.73,19.81 32.73,10.92 35.01,8.64 48.47,8.64 U3.12
SCK
  Bottom 0.305: U2.9 9.16,26.91 7.11,28.96 ICSP.2
SIM_CLK
  Bottom 0.305: U4.3 14.57,16.7 14.57,8.26 17.11,5.71 24.6,5.71 29.17,1.14 39.84,1.14 41.39,2.69 U3.15
SIM_DATA
  Bottom 0.305: U4.7 15.58,16.71 15.58,8.13 17.23,6.48 38.19,6.48 38.59,6.08 U3.17
SIM_RST  (via drill 0.3)
  Top 0.305: v17.23,15.37 17.23,13.59 v17.49,13.34
  Bottom 0.305: v17.49,13.34 17.49,9.4 19.14,7.75 41.87,7.75 42.79,6.83 U3.14 | 16.98,16.89 16.98,16.76 | U4.2 16.97,16.77 16.98,16.76 | 16.98,16.76 16.98,15.66 17.27,15.37 v17.23,15.37
UART_RXD
  Bottom 0.305: U2.21 19.13,32.08 R17.2
UART_TXD
  Bottom 0.305: U2.20 18.33,33.22 18.76,33.66 R18.2
UCAP
  Bottom 0.305: U2.6 8.72,24.51 C15.1
VBAT  (via drill 0.41)
  Top 0.406: 8.73,25.15 J4.+ | 13.72,28.32 13.72,28.07 13.46,27.81 | 8.6,25.02 J4.+ | J4.+ 8.67,25.15 6.22,25.15 4.57,23.5 4.57,15.88 5.26,15.18 7.44,15.18 v7.49,15.24 | 19.43,16 19.56,16.13 | 19.56,16.13 19.56,15.88 | 19.56,15.88 L3.1 | 19.56,15.88 19.55,15.87 L3.1 19.55,15.5 20.07,14.99 20.07,12.83 19.68,12.45 14.35,12.45 v12.19,10.29 9.4,7.49 D2.- 7.49,7.49 6.79,6.79 U1.3 | 19.56,16.13 19.56,18.2 U7.6 | U7.6 U7.5 | U7.6 18.35,18.35 C1.1
  Top 1.016: 8.73,25.15 10.54,25.15 13.72,28.32 v44.2,28.32
  Bottom 0.305: U3.42 v44.19,28.31 v44.2,28.32 v42.8,28.32 v42.79,28.31 U3.41
  Bottom 0.406: v7.49,15.24 11.3,15.24 12.32,14.22 12.32,10.41 v12.19,10.29
VSIM
  Bottom 0.305: C20.1 19.37,8.91 18.38,9.91 18.38,14.1 19.52,15.24 19.51,15.25 19.51,15.49 | U4.1 19.51,15.49 | U3.16 39.99,6.58 39.46,7.11 18.76,7.11 16.6,9.27 16.6,13.72 17.49,14.61 17.74,14.61 18.76,15.62 19.39,15.62 19.51,15.49
VUSB  (via drill 0.41)
  Top 0.406: 3.81,13.97 3.81,20.95 v3.43,21.34 | D1.+ 10.03,15.84 D6.A v10.03,14.1 | v7.49,14.1 3.94,14.1 3.81,13.97 | J5.1 4.25,12.89 3.81,13.34 3.81,13.97
  Bottom 0.305: 10.1,21.34 U2.2 10.15,21.34
  Bottom 0.406: 10.1,21.34 C19.1 v3.43,21.34 | U2.7 12.12,25.31 12.79,24.64 12.79,22.1 12.03,21.34 10.15,21.34 | v10.03,14.1 v7.5,14.1 v7.49,14.1
XTAL3
  Bottom 0.305: U2.16 15.13,31.45 R5.2 14.46,32.12 Y2.1
XTAL4
  Bottom 0.305: U2.17 15.93,31.59 R5.1 16.46,32.12 Y2.3

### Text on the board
tPlace: IIC | A0 | + | - | D7 | D6
bPlace: v1.0 | www.elecrow.com | 32u4 with A7 GPRS/GSM/GPS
